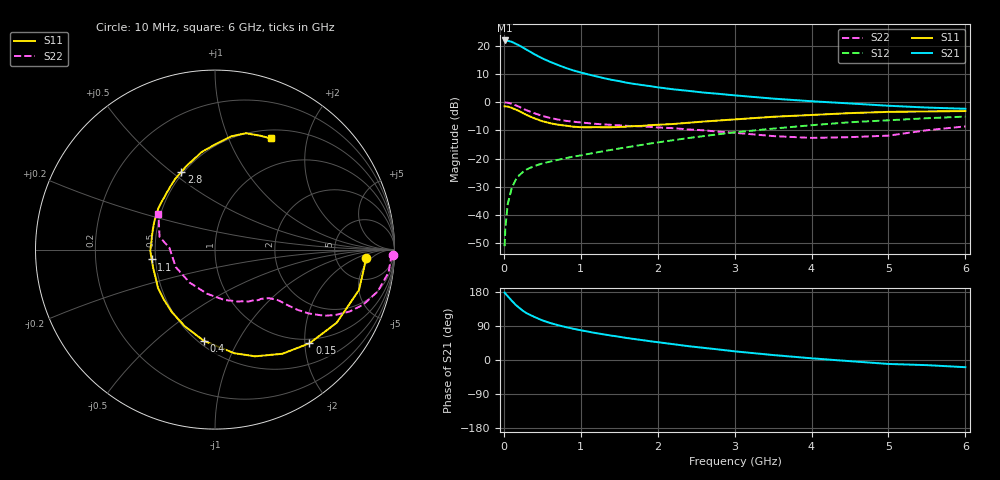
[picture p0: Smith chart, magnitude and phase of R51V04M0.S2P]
! SIEMENS Small Signal Semiconductors
! BFR183
! Si NPN RF Bipolar Junction Transistor in SOT23
! VCE = 1 V  IC = 4 mA
! Common Emitter S-Parameters:  May  1996
# GHz  S  MA  R  50
!  f  S11  S21  S12  S22
! GHz  MAG  ANG  MAG  ANG  MAG  ANG  MAG  ANG
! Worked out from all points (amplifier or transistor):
!   36 points, 10 MHz to 6 GHz, reference 50 ohm
!   highest |S21| = 21.8 dB at 10 MHz (marker M1)
!   |S21| within 3 dB of that: start of sweep to 278.9 MHz
!   unconditionally stable (mu >= 1): 1.068 GHz to 2.896 GHz
!   at 250 MHz: K = 0.37, MSG = 22.0 dB, |S12| = -24.7 dB
!   at 1.4 GHz: K = 1.08, MAG = 10.7 dB, |S12| = -16.9 dB
!   at 6 GHz: K = 0.93, MSG = 1.4 dB, |S12| = -5.1 dB
!   S11 on the Smith chart (normalised r, x): 10 MHz: 10, -3; 150 MHz: 0.91, -2.10; 400 MHz: 0.53, -0.74; 1.1 GHz: 0.48, -0.06; 2.8 GHz: 0.49, +0.54; 6 GHz: 0.61, +1.45
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0.01  0.8416 -3.3  12.35 177.9  0.0028 86.5  0.9898 -1.6
0.02  0.8378 -6.4  12.3 175.1  0.0059 87.4  0.9814 -3.0
0.05  0.8332 -15.7  12.15 168.4  0.0155 80.3  0.9754 -7.5
0.1  0.7911 -31.0  11.76 157.1  0.0292 74.1  0.9363 -14.4
0.15  0.7413 -44.8  10.87 146.3  0.0411 67.5  0.8809 -20.4
0.2  0.6912 -57.1  10.07 137.6  0.0505 62.7  0.8241 -24.8
0.25  0.6353 -69.4  9.235 129.6  0.0581 58.5  0.7634 -28.5
0.3  0.587 -79.5  8.404 123.1  0.0644 55.9  0.7116 -31.2
0.4  0.513 -96.7  7.015 113.4  0.074 51.9  0.6314 -34.3
0.5  0.4593 -111.5  5.942 104.6  0.0817 50.0  0.5703 -36.1
0.6  0.4227 -124.8  5.181 97.8  0.0881 49.7  0.5231 -37.1
0.7  0.3984 -135.7  4.565 92.1  0.0945 49.7  0.4918 -37.8
0.9  0.3663 -154.5  3.65 82.6  0.108 50.1  0.4502 -38.8
1.1  0.3571 -171.2  3.086 74.7  0.1206 51.3  0.4229 -40.6
1.3  0.3571 174.8  2.655 67.6  0.1354 52.3  0.4016 -42.3
1.6  0.3679 158.5  2.202 58.0  0.1584 52.9  0.3792 -46.2
2.2  0.409 132.9  1.684 41.8  0.2109 51.7  0.345 -56.9
2.8  0.4723 113.3  1.397 27.6  0.2705 47.6  0.2985 -72.4
3.5  0.549 97.7  1.152 13.1  0.3389 40.0  0.2498 -100.3
4.5  0.6374 81.9  0.946 -3.1  0.4394 27.7  0.2392 -155.8
5.5  0.6824 68.5  0.8 -13.6  0.5181 15.1  0.3168 167.1
6  0.6935 63.2  0.761 -19.0  0.5528 6.9  0.3713 148.1
